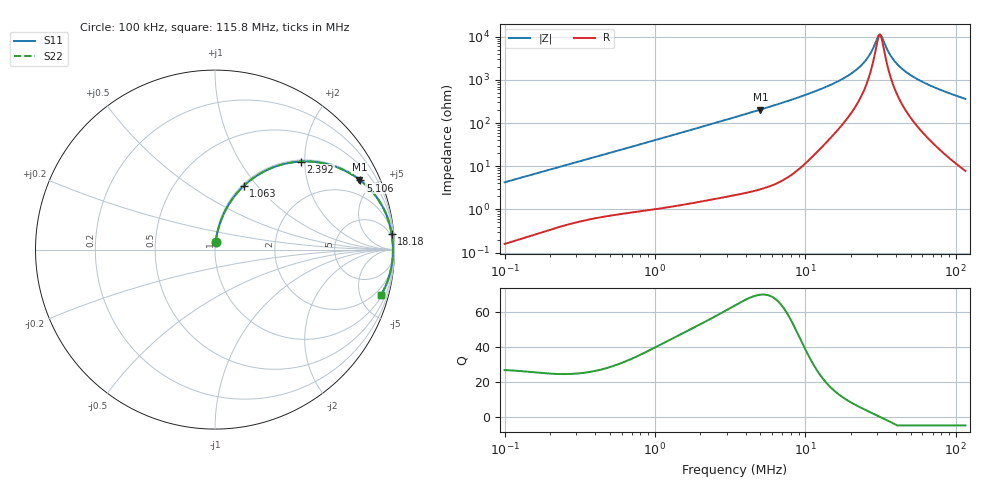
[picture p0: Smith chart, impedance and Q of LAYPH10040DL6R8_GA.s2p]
! LAYPH10040DL6R8_GA  S-PARAMETER MODEL  ( General Type )
! Model Generated by TAIYO YUDEN Corporation (http://www.ty-top.com)
! Version 1.0
! TAIYO YUDEN Control No. 180920NI43SB-FBB
! Copyright(c) 2018 TAIYO YUDEN CO.,LTD. All Rights Reserved.
! Product Description (link to TY-COMPAS)
! https://ds.yuden.co.jp/TYCOMPAS/or/detail?pn=LAYPH10040DL6R8NGA&u=M
! Products Name : Inductors
! Characteristics :
!  Inductance : 6.8 uH , SRF(min) : -Hz , DC Resistance(max) : 0.031 Ohm
!  Rated Current : Saturation :4.3 A , Temp Rise : 2.3 A (25 degC)
!  Case Size : 10.1 x 10.0 / 0.398 x 0.394 [mm/inch] , Thickness : 4 / 0.157 [mm/inch]
!  (Conditions: Temperature = 25 degC , DC Bias Current/Voltage = 0A / 0V)
! External Node Assignments :
!  1  o---GGG---o  2
! GND o---------o GND
! Frequency Range : 0.1MHz  -  115.823372MHz  [ 402 STEP ]
# MHz S RI R 50
! Freq[MHz].  S11 Real  S11 Imag  S21 Real  S21 Imag  S12 Real  S12 Imag  S22 Real  S22 Imag
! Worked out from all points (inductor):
!   401 points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, 100 kHz to 115.8 MHz, reference 50 ohm
!   read as one part in series: L = 6.74 uH near 103.6 kHz
!   highest Q = 69.9 at 5.017 MHz (marker M1), where L = 6.5 uH
!   self-resonance near 30.86 MHz
!   S11 on the Smith chart (normalised r, x): 100 kHz: 1.00, +0.09; 1.063 MHz: 1.02, +0.85; 2.392 MHz: 1.03, +1.92; 5.106 MHz: 1.06, +4.17; 18.18 MHz: 3, +22; 115.8 MHz: 1.16, -7.26
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0.1  0.00339 0.0424  0.9966 -0.0424  0.9966 -0.0424  0.00339 0.0424
0.325976  0.0228 0.1306  0.9772 -0.1306  0.9772 -0.1306  0.0228 0.1306
0.637157  0.069 0.2382  0.931 -0.2382  0.931 -0.2382  0.069 0.2382
1.062605  0.1604 0.3549  0.8396 -0.3549  0.8396 -0.3549  0.1604 0.3549
1.538938  0.2799 0.4387  0.7201 -0.4387  0.7201 -0.4387  0.2799 0.4387
2.391709  0.4793 0.4908  0.5207 -0.4908  0.5207 -0.4908  0.4793 0.4908
3.463838  0.6582 0.4666  0.3418 -0.4666  0.3418 -0.4666  0.6582 0.4666
5.01657  0.8042 0.3897  0.1958 -0.3897  0.1958 -0.3897  0.8042 0.3897
5.10583  0.8099 0.3853  0.1901 -0.3853  0.1901 -0.3853  0.8099 0.3853
11.09389  0.9579 0.1855  0.0421 -0.1855  0.0421 -0.1855  0.9579 0.1855
18.17815  0.9838 0.0871  0.0162 -0.0871  0.0162 -0.0871  0.9838 0.0871
21.68426  0.9879 0.0575  0.0121 -0.0575  0.0121 -0.0575  0.9879 0.0575
24.97011  0.9899 0.0349  0.0101 -0.0349  0.0101 -0.0349  0.9899 0.0349
27.27206  0.9907 0.0211  0.00931 -0.0211  0.00931 -0.0211  0.9907 0.0211
30.85563  0.9912 0.002  0.0088 -0.002  0.0088 -0.002  0.9912 0.002
31.40465  0.9912 -0.000725  0.00878 0.000725  0.00878 0.000725  0.9912 -0.000725
32.53216  0.9912 -0.00618  0.00878 0.00618  0.00878 0.00618  0.9912 -0.00618
36.16345  0.9909 -0.0226  0.00913 0.0226  0.00913 0.0226  0.9909 -0.0226
42.38432  0.9893 -0.0479  0.0107 0.0479  0.0107 0.0479  0.9893 -0.0479
53.30631  0.9846 -0.0865  0.0154 0.0865  0.0154 0.0865  0.9846 -0.0865
74.52619  0.9697 -0.1506  0.0303 0.1506  0.0303 0.1506  0.9697 -0.1506
115.8234  0.9248 -0.2532  0.0752 0.2532  0.0752 0.2532  0.9248 -0.2532
